TYPE E_NCHomeStep :
(
	STATE_HOME_STANDSTILL		:= 1,	(* 回零待命 *)  
	STATE_HOME_DISABLELIMIT		:= 2,	(* 回零，禁用CoE限位监控 *)                             
	STATE_HOME_ABSOLUTESWITCH	:= 3, 	(* 原点回零中 *)	                            
	STATE_HOME_LIMITSWITCH		:= 4, 	(* 限位回零中 *)	                            
	STATE_HOME_ZPULSE			:= 5,	(* Z脉冲回零中 *)                            
	STATE_HOME_BLOCK_1			:= 6,	(* 堵转回零中1 *)    
	STATE_HOME_BLOCK_2			:= 7,	(* 堵转回零中1 *)
    STATE_HOME_BLOCK_3			:= 8,	(* 堵转回零中1 *)                                             
	STATE_HOME_ABORTING			:= 9,	(* 终止回零动作 *)                            
	STATE_HOME_FINISH			:= 10, 	(* 结束回零，走到0位置中 *)                            
	STATE_HOME_ENABLELIMIT		:= 11,  (* 启用CoE驱动器限位监控 *)                          
	STATE_CLEAR_POSITION		:= 12,	(* 设置当前位置 *)   
    STATE_CLEAR_POSITION_1		:= 13,	(* 设置当前位置 *)                                                
	STATE_HOME_ADS_RESET		:= 14,  (* 零点偏置回零 - 复位回零完成信号 *)                          
	STATE_HOME_ADS1				:= 15,	(* 零点偏置回零 - 清空偏置1 *)                            
	STATE_HOME_ADS2				:= 16,	(* 零点偏置回零 - 清空偏置2 *)                            
	STATE_HOME_ADS3				:= 17,	(* 零点偏置回零 - 写偏置1 *)                           
	STATE_HOME_ADS4				:= 18,  (* 零点偏置回零 - 写偏置2 *)                         
	STATE_HOME_ADS_FINISH		:= 19,  (* 零点偏置回零 - 写回零完成信号 *)  
	STATE_HOME_ERROR			:= 48,  (* 回零错误 *) 
	STATE_HOME_DONE				:= 49  (* 回零错误 *) 
);
END_TYPE
